|Texas Instruments Incorporated
|LCD GAMMA BUFFERS with I2C INTERFACE
|Programmable Voltage Source
|   with Memory
| Marketing part#   Voltage Range   Package-type   #pins
|BUF01900AIDRCR   2.0V - 5V   SON   10-pin
|BUF01900AIDRCRG4   2.0V - 5V   SON   10-pin
|BUF01900AIDRCT   2.0V - 5V   SON   10-pin
|BUF01900AIDRCTG4   2.0V - 5V   SON   10-pin
|BUF01900AIPW   2.0V - 5V   TSSOP   8-pin
|BUF01900AIPWG4   2.0V - 5V   TSSOP   8-pin
|BUF01900AIPWR   2.0V - 5V   TSSOP   8-pin
|BUF01900AIPWRG4   2.0V - 5V   TSSOP   8-pin
|BUF01901AIDRCR   2.0V - 5V   SON   10-pin
|BUF01901AIDRCRG4   2.0V - 5V   SON   10-pin
|BUF01901AIDRCT   2.0V - 5V   SON   10-pin
|BUF01901AIDRCTG4   2.0V - 5V   SON   10-pin
|BUF01901AIPW   2.0V - 5V   TSSOP   8-pin
|BUF01901AIPWG4   2.0V - 5V   TSSOP   8-pin
|BUF01901AIPWR   2.0V - 5V   TSSOP   8-pin
|BUF01901AIPWRG4   2.0V - 5V   TSSOP   8-pin
|Programmable Reference Generator
|   and 400mA VCOM Driver
| Marketing part#   Voltage Range   Package-type   #pins
|BUF08800AIPWRP   2.0V - 5.5V   HTSSOP   2O-pin
|BUF08800AIPWPRG4   2.0V - 5.5V   HTSSOP   2O-pin
|Programmable Gamma-Voltage Generator and
|   VCOM Calibrator with Integrated Two-Bank Memory
| Marketing part#   Voltage Range   Package-type   #pins
|BUF08821AIPWPR   2.0V - 5V   HTSSOP   20-pin
|BUF08821AIPWPRG4   2.0V - 5V   HTSSOP   20-pin
|BUF08821BIPWPR   2.0V - 5V   HTSSOP   20-pin
|Programmable Gamma-Voltage Generator and
|   High Slew Rate VCOM with Integrated Two-Bank Memory
| Marketing part#   Voltage Range   Package-type   #pins
|BUF08832AIPWR   2.0V - 5V   HTSSOP   20-pin
|REFERENCE VOLTAGE GENERATOR
|   for LCD GAMMA CORRECTION
| Marketing part#   Voltage Range   Package-type   #pins
|BUF12800AIPWP   2.3V - 5.5V   HTSSOP   24-pin
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[IBIS Ver]   4.0
[File name]   gammabuf_i2c_1.ibs
[File Rev]   1.0
[Date]   xx/xx/20xx
[Source]   Texas Instruments Incorporated.
   Analog-eLab, HPA
   12500 TI Blvd
   Dallas, TX -75243
   For Support e-mail: elab_ibis@list.ti.com
[Notes]   Revision History:
   1.0: xx/xx/20xx
   - Initial version of the model
   - Initial Model generated from simulations in TISPICED
   - Model not matched to measurements
   - Ignore warnings related to min and max values of ccomp,
   The device process of these products is CMOS. The ccomp
   values are based on PVT variations as seen in simulations
[Disclaimer]
 This product is designed as an aid for customers of Texas Instruments.
 No warranties, either expressed or implied, with respect to this third
 party software (if any) or with respect to its fitness for any
 particular purpose is claimed by Texas Instruments or the author. The
 software (if any) is provided solely on an "as is" basis. The entire
 risk as to its quality and performance is with the customer
[Copyright] (C) Copyright 2009 Texas Instruments Incorporated.
   All rights reserved.
|   COMPONENTS
|   BUF01900 and BUF01901
|   10-pin SON and
|   8-pin TSSOP
[Component]   BUF01900drc
[Manufacturer] TI
[Package]   | DRC - SON package
|   typ   min   max
R_pkg   3.823E-02   3.527E-02   4.189E-02
L_pkg   9.698E-01nH 8.843E-01nH 1.074E+00nH
C_pkg   1.557E-01pF 1.479E-01pF 1.641E-01pF
[Pin] signal_name  model_name  R_pin  L_pin C_pin
1   VS   TERM   0.04189  1.07368nH  0.15081pF
2   VCOM   TERM   0.03919  0.99734nH  0.16413pF
3   BIAS   TERM   0.03585  0.91009nH  0.15908pF
4   GND   TERM   0.03584  0.91051nH  0.15920pF
5   DGND   GND   0.03970  1.01644nH  0.14881pF
6   VSD   POWER   0.03969  1.00670nH  0.14790pF
7   A1   AX   0.03597  0.90325nH  0.15830pF
8   A0   AX   0.03527  0.88428nH  0.15683pF
9   SCL   SCL   0.03736  0.93956nH  0.16069pF
10   SDA   SDA   0.04158  1.05644nH  0.15090pF
[Component]   BUF01901drc
[Manufacturer] TI
[Package]   | DRC - SON package
|   typ   min   max
R_pkg   3.823E-02   3.527E-02   4.189E-02
L_pkg   9.698E-01nH 8.843E-01nH 1.074E+00nH
C_pkg   1.557E-01pF 1.479E-01pF 1.641E-01pF
[Pin] signal_name  model_name  R_pin  L_pin C_pin
1   VS   TERM   0.04189  1.07368nH  0.15081pF
2   NC   NC   0.03919  0.99734nH  0.16413pF
3   BIAS   TERM   0.03585  0.91009nH  0.15908pF
4   GND   TERM   0.03584  0.91051nH  0.15920pF
5   DGND   GND   0.03970  1.01644nH  0.14881pF
6   VSD   POWER   0.03969  1.00670nH  0.14790pF
7   A1   AX   0.03597  0.90325nH  0.15830pF
8   A0   AX   0.03527  0.88428nH  0.15683pF
9   SCL   SCL   0.03736  0.93956nH  0.16069pF
10   SDA   SDA   0.04158  1.05644nH  0.15090pF
[Component]   BUF01900pw
[Manufacturer] TI
[Package]   | PW - TSSOP package
|   typ   min   max
R_pkg   0.062591   0.037150   0.073530
L_pkg   1.626966nH 1.394880nH 1.756570nH
C_pkg   0.269755pF 0.251340pF 0.287200pF
[Pin] signal_name  model_name  R_pin  L_pin C_pin
1   VS   TERM   0.07353  1.75657nH  0.25134pF
2   VCOM   TERM   0.07062  1.68957nH  0.27022pF
3   BIAS   TERM   0.06990  1.67677nH  0.27175pF
4   GND   GND   0.03715  1.41063nH  0.28561pF
5   VSD   POWER   0.03728  1.39488nH  0.28720pF
6   AO   AX   0.06997  1.67847nH  0.27091pF
7   SCL   SCL   0.06925  1.66247nH  0.26907pF
8   SDA   SDA   0.07303  1.74637nH  0.25194pF
[Component]   BUF01901pw
[Manufacturer] TI
[Package]   | PW - TSSOP package
|   typ   min   max
R_pkg   0.062591   0.037150   0.073530
L_pkg   1.626966nH 1.394880nH 1.756570nH
C_pkg   0.269755pF 0.251340pF 0.287200pF
[Pin] signal_name  model_name  R_pin  L_pin C_pin
1   VS   TERM   0.07353  1.75657nH  0.25134pF
2   VCOM   TERM   0.07062  1.68957nH  0.27022pF
3   BIAS   TERM   0.06990  1.67677nH  0.27175pF
4   GND   GND   0.03715  1.41063nH  0.28561pF
5   VSD   POWER   0.03728  1.39488nH  0.28720pF
6   AO   AX   0.06997  1.67847nH  0.27091pF
7   SCL   SCL   0.06925  1.66247nH  0.26907pF
8   SDA   SDA   0.07303  1.74637nH  0.25194pF
|   BUF08800
|   20-pin HTSSOP
[Component]   BUF08800pwp
[Manufacturer] TI
[Package]   |PWP PowerPAD - HTSSOP package
|   typ   min   max
R_pkg   0.083366   0.036020   0.113300
L_pkg   2.812828nH 2.279060nH 3.506060nH
C_pkg   0.502554pF 0.442270pF 0.611200pF
[Pin] signal_name  model_name  R_pin  L_pin C_pin
1   GND   TERM   0.05117  3.08196nH  0.61120pF
2   GND   TERM   0.03839  2.80189nH  0.58862pF
3   PIN_VCOM   TERM   0.10112  2.77274nH  0.45325pF
4   NIN_VCOM   TERM   0.08933  2.53792nH  0.44984pF
5   VSD   POWER   0.08368  2.42835nH  0.44227pF
6   SCL   SCL   0.08572  2.46946nH  0.44393pF
7   SDA   SDA   0.09375  2.62877nH  0.45376pF
8   A0   AX   0.10656  2.88624nH  0.45703pF
9   LD   AX   0.11330  3.33087nH  0.53501pF
10   GND_DIGITAL  GND   0.09923  3.50606nH  0.57076pF
11   OUT8   TERM   0.09636  3.44966nH  0.56772pF
12   OUT7   TERM   0.11065  3.27837nH  0.53209pF
13   OUT6   TERM   0.10444  2.84424nH  0.45462pF
14   OUT5   TERM   0.09215  2.59717nH  0.45204pF
15   OUT4   TERM   0.08484  2.45196nH  0.44310pF
16   OUT3   TERM   0.08406  2.43535nH  0.44227pF
17   OUT2   TERM   0.09002  2.55122nH  0.45312pF
18   VS   TERM   0.03602  2.27906nH  0.52524pF
29   VS   TERM   0.05477  2.81113nH  0.56717pF
20   VCOM_OUT1   TERM   0.05176  3.11413nH  0.60804pF
|   BUF08821
|   20-pin HTSSOP
[Component]   BUF08821pwp
[Manufacturer] TI
[Package]   |PWP PowerPAD - HTSSOP
|   typ   min   max
R_pkg  7.857E-02   4.440E-03   1.157E-01
L_pkg  2.881nH   2.148nh   3.751nH
C_pkg  0.4867pF   0.4355pF   0.5664pF
[Pin] signal_name  model_name  R_pin  L_pin C_pin
1   VCOM   TERM   0.0943   3.73495nH  0.56644pF
2   OUT1   TERM   0.11572  3.6559nH   0.53542pF
3   OUT2   TERM   0.1058   3.08334nH  0.45933pF
4   OUT3   TERM   0.09101  2.78584nH  0.45405pF
5   OUT4   TERM   0.08024  2.57369nH  0.4409pF
6   VS   TERM   0.04007  2.14752nH  0.47985pF
7   GNDA   TERM   0.04032  2.15429nH  0.48021pF
8   VSD   POWER   0.08785  2.73278nH  0.43769pF
9   SCL   SCL   0.09914  3.31155nH  0.51919pF
10  SDA   SDA   0.09436  3.7505nH   0.56644pF
11  A0   AX   0.09413  3.7459nH   0.56634pF
12  BKSEL  BKSEL   0.09917  3.31215nH  0.51915pF
13  GNDD   GND   0.0886   2.74768nH  0.43549pF
14  OUT5   TERM   0.08388  2.65011nH  0.44421pF
15  VS   TERM   0.0403   2.15648nH  0.48406pF
16  GNDA   TERM   0.04018  2.14797nH  0.48136pF
17  OUT6   TERM   0.08113  2.59194nH  0.44219pF
18  OUT7   TERM   0.09239  2.81764nH  0.44292pF
19  OUT8   TERM   0.09836  3.3102nH   0.50987pF
20  NC   NC   0.00444  2.20055nH  0.46896pF
|   BUF08832
|   20-pin HTSSOP
[Component]   BUF08832pwp
[Manufacturer] TI
[Package]   |PWP PowerPAD
|   typ   min   max
R_pkg   0.076857   0.039770   0.102370
L_pkg   2.626745nH 1.930650nH 3.555430nH
C_pkg   0.485737pF 0.428810pF 0.605160pF
[Pin] signal_name  model_name  R_pin  L_pin C_pin
1   VCOM   TERM   0.05042  3.04264nH  0.60516pF
2   GNDA   TERM   0.05018  2.59932nH  0.55292pF
3   OUT1   TERM   0.08640  2.48404nH  0.43167pF
4   OUT2   TERM   0.08011  2.35742nH  0.43743pF
5   OUT3   TERM   0.07106  2.18295nH  0.42923pF
6   OUT4   TERM   0.07160  2.19536nH  0.42994pF
7   VS   TERM   0.04181  1.99239nH  0.47169pF
8   VSD   POWER   0.08779  2.51644nH  0.43281pF
9   SCL   SCL   0.09912  3.05057nH  0.51581pF
10   SDA   SDA   0.09522  3.42676nH  0.56413pF
11   A0   AX   0.09605  3.44316nH  0.56535pF
12   BKSEL   BKSEL   0.10053  3.07837nH  0.51794pF
13   GNDD   GND   0.08776  2.51564nH  0.43344pF
14   GNDA   TERM   0.03977  1.93065nH  0.46812pF
15   OUT5   TERM   0.07012  2.16596nH  0.42881pF
16   OUT6   TERM   0.07438  2.24625nH  0.43340pF
17   OUT7   TERM   0.08693  2.48972nH  0.44582pF
18   OUT8   TERM   0.09541  2.65994nH  0.44052pF
19   VS   TERM   0.05010  2.60188nH  0.54142pF
20   VCOM_FB   TERM   0.10237  3.55543nH  0.56912pF
|   BUF12800
|   24-pin HTSSOP
[Component]   BUF12800pwp
[Manufacturer] TI
[Package]   |PWP PowerPAD
|   typ   min   max
R_pkg   0.092542   0.000570   0.125530
L_pkg   3.045318nH 0.768720nH 4.217140nH
C_pkg   0.577033pF 0.495830pF 1.541880pF
[Pin] signal_name  model_name  R_pin  L_pin C_pin
1   VS   TERM   0.12054  4.21714nH  0.62518pF
2   VS   TERM   0.11569  3.39849nH  0.53273pF
3   REFH   TERM   0.09758  3.04447nH  0.52807pF
4   VSD   POWER   0.08787  2.85728nH  0.51930pF
5   SCL   SCL   0.07872  2.66808nH  0.50144pF
6   SDA   SDA   0.07474  2.58534nH  0.49606pF
7   A0   AX   0.07465  2.58525nH  0.49583pF
8   LD   AX   0.07845  2.66687nH  0.50088pF
9   GNDD   GND   0.08742  2.85455nH  0.51717pF
10   REFL   TERM   0.09196  2.94101nH  0.51936pF
11   GNDA   TERM   0.12452  3.57980nH  0.54191pF
12   GNDA   TERM   0.11704  4.15037nH  0.62498pF
13   OUTA   TERM   0.10768  3.96643nH  0.61983pF
14   OUTB   TERM   0.12351  3.56040nH  0.55205pF
15   OUTC   TERM   0.10169  3.13256nH  0.53870pF
16   OUTD   TERM   0.08976  2.90101nH  0.52272pF
17   OUTE   TERM   0.07987  2.69509nH  0.50404pF
18   OUTF   TERM   0.07464  2.58484nH  0.49683pF
19   OUTG   TERM   0.07496  2.59004nH  0.49720pF
20   OUTH   TERM   0.08112  2.71521nH  0.50555pF
21   OUTI   TERM   0.09163  2.93136nH  0.52480pF
22   OUTJ   TERM   0.10346  3.16007nH  0.54068pF
23   OUTK   TERM   0.12553  3.59178nH  0.55415pF
24   OUTL   TERM   0.10994  3.98679nH  0.62449pF
|   BUF16820
|   32-pin HTSSOP
[Component]   BUF16820dap
[Manufacturer] TI
[Package]   |HTSSOP PowerPAD
|   typ   min   max
R_pkg   0.094521   0.001790   0.126830
L_pkg   3.001572nH 0.917530nH 4.064830nH
C_pkg   0.494037pF 0.270370pF 0.696050pF
[Pin] signal_name  model_name  R_pin  L_pin C_pin
1   VCOM2   TERM   0.08279  3.90977nH  0.68574pF
2   REFH   TERM   0.08451  3.47476nH  0.66524pF
3   OUT1   TERM   0.08790  3.11205nH  0.58559pF
4   OUT2   TERM   0.10765  3.14464nH  0.50531pF
5   OUT3   TERM   0.12416  3.05611nH  0.40478pF
6   OUT4   TERM   0.11289  2.83628nH  0.39291pF
7   OUT5   TERM   0.10539  2.66296nH  0.38412pF
8   OUT6   TERM   0.10164  2.59101nH  0.37906pF
9   GNDA   TERM   0.10211  2.60110nH  0.37958pF
10   VS   TERM   0.10658  2.68895nH  0.38417pF
11   OUT7   TERM   0.11157  2.81534nH  0.39003pF
12   OUT8   TERM   0.12245  3.02917nH  0.40199pF
13   OUT9   TERM   0.10387  3.16179nH  0.50312pF
14   REFH_OUT  TERM   0.08586  3.13814nH  0.60097pF
15   VSD   POWER   0.08296  3.49951nH  0.66718pF
16   SCL   SCL   0.08055  3.96757nH  0.69457pF
17   SDA   SDA   0.09044  4.06483nH  0.69605pF
18   A0   AX   0.09424  3.66921nH  0.68207pF
19   LD   AX   0.09979  3.34902nH  0.60477pF
20   GNDD   GND   0.10789  3.15807nH  0.50525pF
21   OUT10   TERM   0.10968  2.77914nH  0.38647pF
22   OUT11   TERM   0.10289  2.64529nH  0.38088pF
23   OUT12   TERM   0.10140  2.58686nH  0.37944pF
24   OUT13   TERM   0.10378  2.63198nH  0.38098pF
25   VS   TERM   0.10817  2.71658nH  0.38611pF
26   GNDA   TERM   0.11717  2.89126nH  0.39659pF
27   OUT14   TERM   0.12683  3.10789nH  0.40041pF
28   NC   NC   0.00179  0.91753nH  0.27037pF
29   NC   NC   0.00253  1.34491nH  0.38564pF
30   REFL_OUT  TERM   0.08790  3.11247nH  0.57857pF
31   REFL   TERM   0.08450  3.47517nH  0.66534pF
32   VCOM1   TERM   0.08280  3.91093nH  0.68587pF
|   BUF16821
|   28-pin HTSSOP
[Component]   BUF16821pwp
[Manufacturer] TI
[Package]   |PWP PowerPAD - HTSSOP package
|   typ   min   max
R_pkg   0.101552   0.039420   0.152910
L_pkg   3.114714nH 2.047180nH 4.363310nH
C_pkg   0.504927pF 0.433040pF 0.615400pF
[Pin] signal_name  model_name  R_pin  L_pin C_pin
1   VCOM2   TERM   0.13256  4.26300nH  0.61145pF
2   OUT1   TERM   0.15291  4.24862nH  0.59970pF
3   OUT2   TERM   0.13345  3.51246nH  0.49558pF
4   OUT3   TERM   0.11258  3.10174nH  0.48402pF
5   OUT4   TERM   0.09644  2.78445nH  0.46350pF
6   OUT5   TERM   0.08487  2.56708nH  0.44539pF
7   OUT6   TERM   0.07765  2.42575nH  0.43654pF
8   GNDA   TERM   0.03942  2.04718nH  0.47733pF
9   VS   TERM   0.04012  2.08579nH  0.48456pF
10   OUT7   TERM   0.08361  2.53893nH  0.44984pF
11   OUT8   TERM   0.09645  2.79076nH  0.46238pF
12   OUT9   TERM   0.11515  3.15775nH  0.46989pF
13   VSD   POWER   0.12984  3.80219nH  0.56785pF
14   SCL   SCL   0.12907  4.20986nH  0.60777pF
15   SDA   SDA   0.13688  4.36331nH  0.61540pF
16   A0   AX   0.13883  3.97565nH  0.57857pF
17   BKSEL   BKSEL   0.11484  3.15088nH  0.46955pF
18   GNDD   GND   0.08767  2.61714nH  0.44825pF
19   OUT10   TERM   0.08410  2.54845nH  0.44355pF
20   OUT11   TERM   0.07692  2.42064nH  0.43803pF
21   OUT12   TERM   0.07516  2.37847nH  0.43304pF
22   OUT13   TERM   0.07924  2.45616nH  0.44041pF
23   VS   TERM   0.04564  2.26978nH  0.50068pF
24   GNDA   TERM   0.05104  2.42319nH  0.52327pF
25   OUT14   TERM   0.11207  3.09152nH  0.48573pF
26   OUT15   TERM   0.13288  3.50113nH  0.49501pF
27   OUT16   TERM   0.15221  4.23192nH  0.59954pF
28   VCOM1   TERM   0.13186  4.24818nH  0.61113pF
|   BUF20800 and BUF20820
|   38-pin HTSSOP
[Component]   BUF20800dcp
[Manufacturer] TI
[Package]   |DCP PowerPAD
|   typ   min   max
R_pkg   0.073288   0.005260   0.104970
L_pkg   2.795736nH 1.603620nH 4.377360nH
C_pkg   0.521176pF 0.422720pF 0.736230pF
[Pin] signal_name  model_name  R_pin  L_pin C_pin
1   VCOM_OUT2  TERM   0.10175  4.33591nH  0.68578pF
2   REFH   TERM   0.10160  4.02207nH  0.72391pF
3   NC   NC   0.00699  2.12027nH  0.55627pF
4   NC   NC   0.00526  1.60362nH  0.42517pF
5   OUT1   TERM   0.08790  2.61008nH  0.44023pF
6   OUT2   TERM   0.07873  2.43374nH  0.44294pF
7   OUT3   TERM   0.07101  2.28711nH  0.43287pF
8   OUT4   TERM   0.06547  2.18255nH  0.42592pF
9   OUT5   TERM   0.06294  2.13633nH  0.42272pF
10   OUT6   TERM   0.06381  2.15352nH  0.42425pF
11   GNDA   TERM   0.03583  1.94104nH  0.46522pF
12   VS   TERM   0.03892  2.04826nH  0.47417pF
13   OUT7   TERM   0.07658  2.39852nH  0.44076pF
14   OUT8   TERM   0.08545  2.56935nH  0.45284pF
15   OUT9   TERM   0.09539  2.76249nH  0.45679pF
16   REFOUT   TERM   0.10497  3.30781nH  0.53950pF
17   VSD   POWER   0.10352  3.76251nH  0.66775pF
18   SCL   SCL   0.10315  4.06757nH  0.73600pF
19   SDA   SDA   0.10335  4.37736nH  0.68930pF
20   A0   AX   0.10309  4.37246nH  0.68932pF
21   LD   AX   0.10308  4.06627nH  0.73623pF
22   GNDD   GND   0.10348  3.76161nH  0.66777pF
23   OUT10   TERM   0.10497  3.30781nH  0.53952pF
24   OUT11   TERM   0.09540  2.76249nH  0.45679pF
25   OUT12   TERM   0.08545  2.56945nH  0.45284pF
26   OUT13   TERM   0.07658  2.39852nH  0.44076pF
27   VS   TERM   0.03893  2.05014nH  0.47376pF
28   GNDA   TERM   0.03591  1.94388nH  0.46519pF
29   OUT14   TERM   0.06381  2.15356nH  0.42435pF
30   OUT15   TERM   0.06294  2.13638nH  0.42273pF
31   OUT16   TERM   0.06547  2.18259nH  0.42593pF
32   OUT17   TERM   0.07101  2.28721nH  0.43287pF
33   OUT18   TERM   0.07873  2.43384nH  0.44295pF
34   REFL_OUT   TERM   0.08790  2.61008nH  0.44023pF
35   NC   NC   0.00526  1.60362nH  0.42517pF
36   NC   NC   0.00699  2.12027nH  0.55627pF
37   REFL   TERM   0.10159  4.02177nH  0.72387pF
38   VCOM_OUT1  TERM   0.10175  4.33591nH  0.68575pF
|   BUF20800 and BUF20820
|   38-pin HTSSOP
[Component]   BUF20820dcp
[Manufacturer] TI
[Package]   |DCP PowerPAD
|   typ   min   max
R_pkg   0.073288   0.005260   0.104970
L_pkg   2.795736nH 1.603620nH 4.377360nH
C_pkg   0.521176pF 0.422720pF 0.736230pF
[Pin] signal_name  model_name  R_pin  L_pin C_pin
1   VCOM_OUT2  TERM   0.10175  4.33591nH  0.68578pF
2   REFH   TERM   0.10160  4.02207nH  0.72391pF
3   NC   NC   0.00699  2.12027nH  0.55627pF
4   NC   NC   0.00526  1.60362nH  0.42517pF
5   OUT1   TERM   0.08790  2.61008nH  0.44023pF
6   OUT2   TERM   0.07873  2.43374nH  0.44294pF
7   OUT3   TERM   0.07101  2.28711nH  0.43287pF
8   OUT4   TERM   0.06547  2.18255nH  0.42592pF
9   OUT5   TERM   0.06294  2.13633nH  0.42272pF
10   OUT6   TERM   0.06381  2.15352nH  0.42425pF
11   GNDA   TERM   0.03583  1.94104nH  0.46522pF
12   VS   TERM   0.03892  2.04826nH  0.47417pF
13   OUT7   TERM   0.07658  2.39852nH  0.44076pF
14   OUT8   TERM   0.08545  2.56935nH  0.45284pF
15   OUT9   TERM   0.09539  2.76249nH  0.45679pF
16   REFOUT   TERM   0.10497  3.30781nH  0.53950pF
17   VSD   POWER   0.10352  3.76251nH  0.66775pF
18   SCL   SCL   0.10315  4.06757nH  0.73600pF
19   SDA   SDA   0.10335  4.37736nH  0.68930pF
20   A0   AX   0.10309  4.37246nH  0.68932pF
21   LD   AX   0.10308  4.06627nH  0.73623pF
22   GNDD   GND   0.10348  3.76161nH  0.66777pF
23   OUT10   TERM   0.10497  3.30781nH  0.53952pF
24   OUT11   TERM   0.09540  2.76249nH  0.45679pF
25   OUT12   TERM   0.08545  2.56945nH  0.45284pF
26   OUT13   TERM   0.07658  2.39852nH  0.44076pF
27   VS   TERM   0.03893  2.05014nH  0.47376pF
28   GNDA   TERM   0.03591  1.94388nH  0.46519pF
29   OUT14   TERM   0.06381  2.15356nH  0.42435pF
30   OUT15   TERM   0.06294  2.13638nH  0.42273pF
31   OUT16   TERM   0.06547  2.18259nH  0.42593pF
32   OUT17   TERM   0.07101  2.28721nH  0.43287pF
33   OUT18   TERM   0.07873  2.43384nH  0.44295pF
34   REFL_OUT   TERM   0.08790  2.61008nH  0.44023pF
35   NC   NC   0.00526  1.60362nH  0.42517pF
36   NC   NC   0.00699  2.12027nH  0.55627pF
37   REFL   TERM   0.10159  4.02177nH  0.72387pF
38   VCOM_OUT1  TERM   0.10175  4.33591nH  0.68575pF
|   BUF22821
|   38-pin HTSSOP
[Component]   BUF22821dcp
[Manufacturer] TI
[Package]   |DCP PowerPAD
|   typ   min   max
R_pkg   0.092863   0.042390   0.128010
L_pkg   3.152992nH 2.128800nH 4.176860nH
C_pkg   0.548287pF 0.442640pF 0.741830pF
[Pin] signal_name  model_name  R_pin  L_pin C_pin
1   VCOM_OUT2  TERM   0.09207  4.14901nH  0.68142pF
2   STATINH   TERM   0.10220  4.03357nH  0.74183pF
3   OUT21   TERM   0.11404  3.95837nH  0.69300pF
4   OUT22   TERM   0.12801  3.74822nH  0.57409pF
5   OUT1   TERM   0.11638  3.16228nH  0.48143pF
6   OUT2   TERM   0.10562  2.95244nH  0.47754pF
7   OUT3   TERM   0.09602  2.76671nH  0.46398pF
8   OUT4   TERM   0.08808  2.61342nH  0.45333pF
9   OUT5   TERM   0.08238  2.50499nH  0.44583pF
10   OUT6   TERM   0.07951  2.45061nH  0.44264pF
11   GNDA   TERM   0.04244  2.13052nH  0.48664pF
12   VS   TERM   0.04342  2.16394nH  0.49368pF
13   OUT7   TERM   0.08676  2.59302nH  0.45500pF
14   OUT8   TERM   0.09431  2.73945nH  0.46194pF
15   OUT9   TERM   0.10359  2.92089nH  0.46352pF
16   STATOUTH   TERM   0.11339  3.47151nH  0.54793pF
17   VSD   POWER   0.09383  3.57481nH  0.65776pF
18   SCL   SCL   0.09310  3.87287nH  0.72464pF
19   SDA   SDA   0.09299  4.17686nH  0.67802pF
20   A0   AX   0.09224  4.16256nH  0.67744pF
21   BKSEL   BKSEL   0.09250  3.86147nH  0.72432pF
22   GNDD   GND   0.09392  3.57651nH  0.65907pF
23   OUT10   TERM   0.10944  3.39451nH  0.54458pF
24   OUT11   TERM   0.10029  2.85659nH  0.45921pF
25   OUT12   TERM   0.09154  2.68585nH  0.45818pF
26   OUT13   TERM   0.08473  2.55372nH  0.45211pF
27   VS   TERM   0.04291  2.14887nH  0.49173pF
28   GNDA   TERM   0.04239  2.12880nH  0.48654pF
29   OUT14   TERM   0.08021  2.46361nH  0.44365pF
30   OUT15   TERM   0.08415  2.53869nH  0.44793pF
31   OUT16   TERM   0.09047  2.65932nH  0.45632pF
32   OUT17   TERM   0.09902  2.82441nH  0.46794pF
33   OUT18   TERM   0.10905  3.01884nH  0.47925pF
34   STATOUTL   TERM   0.11553  3.14578nH  0.47744pF
35   OUT19   TERM   0.12702  3.72902nH  0.57263pF
36   OUT20   TERM   0.11299  3.93797nH  0.69162pF
37   STATINL   TERM   0.10118  4.01377nH  0.74049pF
38   VCOM1   TERM   0.09107  4.12991nH  0.68025pF
|   MODELS
[Model Selector]  SCL
SCL_33   3V digital input
SCL_5   5V digital input
[Model Selector]  AX
AX_33   3V digital input
AX_5   5V digital input
[Model Selector]  BKSEL
BKSEL_33   3V digital input
BKSEL_5   5V digital input
[Model Selector]  SDA_400
SDA_400_33  3V digital output
SDA_400_5  5V digital output
[Model Selector]  SDA
SDA_3400_33  3V digital output
SDA_3400_5  5V digital output
|   TERM Model
[Model] TERM
Model_type Terminator
C_comp   0   0   0
| variable   typ   min   max
[Voltage Range]   3.0V   2.0V   5.5V
[POWER Clamp Reference]  3.0V   2.0V   5.5V
[GND Clamp Reference]   0.0V   0.0V   0.0V
|Operating Temperature
[Temperature Range]   27   85   -40
| Models and submodels in the file (11): TERM (Terminator), SCL_33 (Input), SCL_5 (Input), AX_33 (Input), AX_5 (Input), BKSEL_33 (Input), BKSEL_5 (Input), SDA_400_33 (I/O_open_drain), SDA_400_5 (I/O_open_drain), SDA_3400_33 (I/O_open_drain), SDA_3400_5 (I/O_open_drain)
